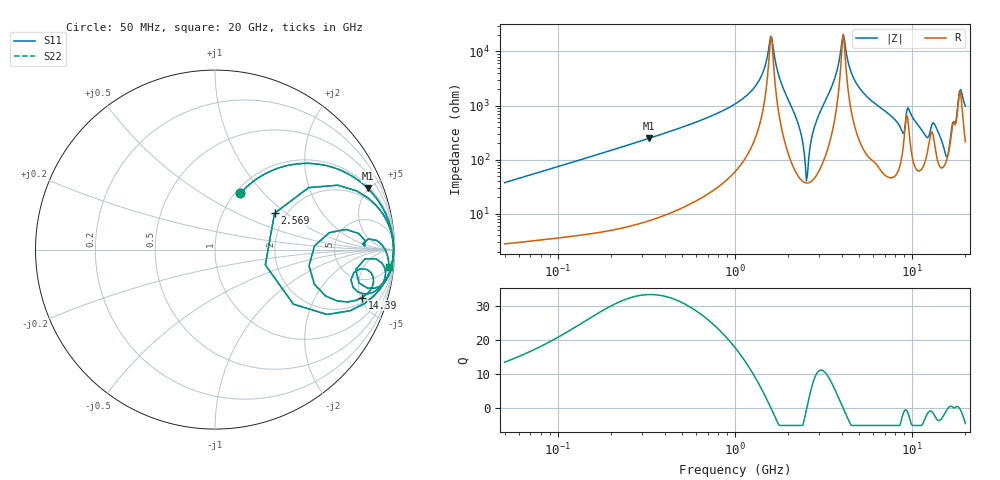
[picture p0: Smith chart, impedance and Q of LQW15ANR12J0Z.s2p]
!Murata Part Number: LQW15ANR12J0Z
!These Parameters are Measured in Series Mode Connection
!  o--[Z]--o
!Port1  Port2
!  o-------o
!Freq. Start=50[MHz] Stop=20[GHz], 401[Steps]
# Hz S RI R 50
!Freq.(Hz) S11(Real) S11(Imag) S21(Real) S21(Imag) S12(Real) S12(Imag) S22(Real) S22(Imag)
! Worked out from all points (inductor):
!   401 points, 50 MHz to 20 GHz, reference 50 ohm
!   read as one part in series: L = 119 nH near 51.52 MHz
!   highest Q = 33.4 at 325.2 MHz (marker M1), where L = 120 nH
!   self-resonance near 1.591 GHz
!   S11 on the Smith chart (normalised r, x): 50 MHz: 1.06, +0.75; 2.569 GHz: 1.74, +0.83; 14.39 GHz: 2.47, -5.14; 20 GHz: 5, -19
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5e7  0.1414 0.3134  0.8586 -0.3134  0.8586 -0.3134  0.1414 0.3134
1.364002e8  0.5062 0.4804  0.4938 -0.4804  0.4938 -0.4804  0.5062 0.4804
3.251725e8  0.851 0.3414  0.149 -0.3414  0.149 -0.3414  0.851 0.3414
3.721004e8  0.8827 0.3071  0.1173 -0.3071  0.1173 -0.3071  0.8827 0.3071
1e9  0.9863 0.0916  0.0137 -0.0916  0.0137 -0.0916  0.9863 0.0916
1.349283e9  0.9939 0.0363  0.00613 -0.0363  0.00613 -0.0363  0.9939 0.0363
1.590961e9  0.995 0.00126  0.00502 -0.00126  0.00502 -0.00126  0.995 0.00126
2.211938e9  0.9579 -0.1577  0.0421 0.1577  0.0421 0.1577  0.9579 -0.1577
2.419936e9  0.7527 -0.3408  0.2473 0.3408  0.2473 0.3408  0.7527 -0.3408
2.569357e9  0.3316 0.2021  0.6684 -0.2021  0.6684 -0.2021  0.3316 0.2021
2.728004e9  0.8538 0.287  0.1462 -0.287  0.1462 -0.287  0.8538 0.287
3.626126e9  0.9934 0.0332  0.00664 -0.0332  0.00664 -0.0332  0.9934 0.0332
4.087748e9  0.9952 -2.96e-05  0.00483 2.96e-05  0.00483 2.96e-05  0.9952 -2.96e-05
4.89267e9  0.9935 -0.0401  0.00645 0.0401  0.00645 0.0401  0.9935 -0.0401
7.442007e9  0.9698 -0.1402  0.0302 0.1402  0.0302 0.1402  0.9698 -0.1402
8.774992e9  0.8501 -0.2149  0.1499 0.2149  0.1499 0.2149  0.8501 -0.2149
9.600142e9  0.9437 -0.0974  0.0563 0.0974  0.0563 0.0974  0.9437 -0.0974
1.183995e10  0.8252 -0.246  0.1748 0.246  0.1748 0.246  0.8252 -0.246
1.438523e10  0.8195 -0.2674  0.1805 0.2674  0.1805 0.2674  0.8195 -0.2674
1.573793e10  0.5239 -0.0901  0.4761 0.0901  0.4761 0.0901  0.5239 -0.0901
1.855685e10  0.9491 -0.00205  0.0509 0.00205  0.0509 0.00205  0.9491 -0.00205
2e10  0.9686 -0.095  0.0314 0.095  0.0314 0.095  0.9686 -0.095
